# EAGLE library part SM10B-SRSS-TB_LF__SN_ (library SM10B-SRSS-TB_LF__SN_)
JST (JAPAN SOLDERLESS TERMINALS) - SM10B-SRSS-TB(LF)(SN) - HEADER, R/A, 10WAY Source: Datasheet
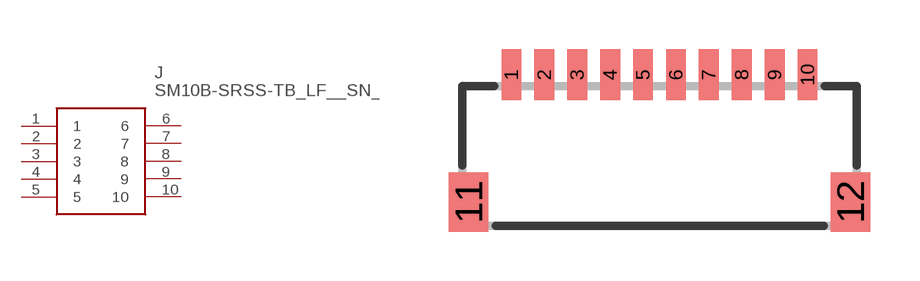
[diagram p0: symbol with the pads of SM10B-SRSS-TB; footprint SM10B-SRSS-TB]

Designator prefix J

## SM10B-SRSS-TB_LF__SN_ (Arrow_Part_Number: SM10B-SRSS-TB(LF)(SN); Arrow_Price-Stock: https://www.arrow.com/en/products/sm10b-srss-tb-lf-sn/jst-manufacturing?utm_currency=USD&region=europe; Description: JST (JAPAN SOLDERLESS TERMINALS) - SM10B-SRSS-TB(LF)(SN) - HEADER, R/A, 10WAY; Height: mm; Manufacturer_Name: JST (JAPAN SOLDERLESS TERMINALS); Manufacturer_Part_Number: SM10B-SRSS-TB(LF)(SN); Mouser_Part_Number: 306-SM10BSRSSTBLFSN; Mouser_Price-Stock: https://www.mouser.co.uk/ProductDetail/JST-Commercial/SM10B-SRSS-TBLFSN?qs=QpmGXVUTftHkZAI%2F8hE40w%3D%3D)  [SM10B-SRSS-TB]
1  1
2  2
3  3
4  4
5  5
6  6
7  7
8  8
9  9
10  10

## Footprint SM10B-SRSS-TB (pad centres in mm)
SM10B-SRSS-TB
smd 0.6 x 1.55: 1 1.5,0.342; 2 2.5,0.342; 3 3.5,0.342; 4 4.5,0.342; 5 5.5,0.342; 6 6.5,0.342; 7 7.5,0.342; 8 8.5,0.342; 9 9.5,0.342; 10 10.5,0.342
smd 1.2 x 1.8: 11 0.2,-3.533; 12 11.8,-3.533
